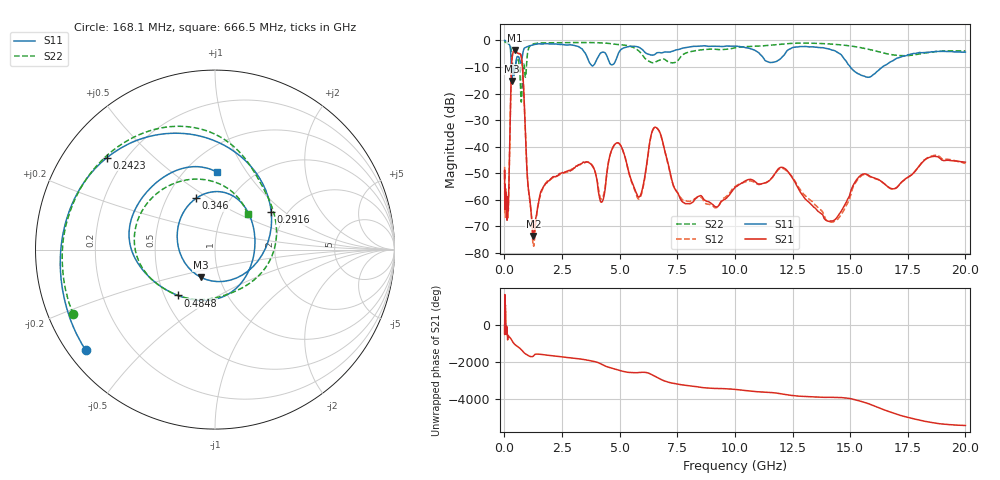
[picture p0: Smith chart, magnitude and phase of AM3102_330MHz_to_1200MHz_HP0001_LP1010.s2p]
! Date/Time: Tue, Sep 11, 2018 5:10 PM
! Network Analyzer: Agilent Technologies E8362B Rev: A.07.50.63
! Sweep from 0.010 to 20.000 GHz, 1601 Points, Sweep Type: LOG
! Power Supply: 4.950 V, 0.001 A
# Hz S DB R 50
!freq MagS11 AngS11 MagS21 AngS21 MagS12 AngS12 MagS22 AngS22
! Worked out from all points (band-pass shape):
!   1601 points, 10 MHz to 20 GHz, reference 50 ohm
!   highest |S21| = -3.62 dB at 443 MHz (marker M1); lowest = -73.7 dB at 1.26 GHz (marker M2)
!   |S21| within 3 dB of the highest: 331.2 MHz to 744.7 MHz (413.5 MHz wide, 76.9 % of centre)
!   lowest |S11| = -15.2 dB at 316.2 MHz (marker M3), VSWR 1.42, Z = 40.9 - j13.1 ohm
!   |S11| at or under -10 dB: 296 MHz to 350.6 MHz (54.65 MHz wide, 16.9 % of centre); 366.7 MHz to 479.5 MHz (112.8 MHz wide, 26.7 % of centre); 15.01 GHz to 16.4 GHz (1.395 GHz wide, 8.88 % of centre)
!   |S22| runs from -23.2 to -0.3 dB; largest |S21 - S12| = 0.012
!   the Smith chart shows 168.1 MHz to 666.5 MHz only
!   S11 on the Smith chart (normalised r, x): 168.1 MHz: 0.05, -0.34; 242.3 MHz: 0.13, +0.36; 291.6 MHz: 1.66, +0.82; 346 MHz: 0.70, +0.44; 484.8 MHz: 0.59, -0.33; 666.5 MHz: 0.70, +0.74
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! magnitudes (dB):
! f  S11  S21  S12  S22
! 10 MHz  0.0  -51.8  -47.6  -0.3
! 35.55 MHz  0.0  -62.2  -60.7  -0.5
! 126.4 MHz  -0.4  -63.5  -65.3  -1.0
! 168.1 MHz  -0.8  -63.1  -63.7  -1.2
! 242.3 MHz  -2.0  -34.8  -34.8  -1.8
! 291.6 MHz  -8.5  -14.2  -14.3  -3.6
! 316.2 MHz  -15.2  -8.3  -8.3  -6.0
! 346 MHz  -10.3  -5.7  -5.8  -8.2
! 443 MHz  -11.9  -3.6  -3.7  -10.8
! 447.2 MHz  -11.7  -3.6  -3.7  -10.6
! 484.8 MHz  -9.7  -3.8  -3.8  -8.9
! 666.5 MHz  -7.3  -5.0  -5.0  -11.5
! 1.26 GHz  -1.6  -73.7  -77.4  -1.3
! 1.59 GHz  -1.3  -56.9  -57.5  -0.9
! 4.23 GHz  -4.5  -60.9  -59.7  -0.9
! 4.878 GHz  -6.5  -38.6  -38.7  -1.5
! 5.652 GHz  -2.2  -55.9  -56.4  -2.9
! 6.58 GHz  -4.9  -32.8  -32.9  -8.0
! 7.92 GHz  -2.6  -61.5  -60.6  -4.6
! 12.03 GHz  -6.4  -47.8  -48.2  -1.4
! 14.21 GHz  -3.6  -68.0  -68.5  -1.4
! 20 GHz  -4.4  -45.9  -46.4  -3.9
